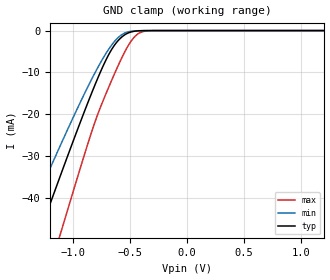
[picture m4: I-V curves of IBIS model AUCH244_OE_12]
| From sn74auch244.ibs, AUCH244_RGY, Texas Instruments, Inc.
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[Model]   AUCH244_OE_12
Model_type  Input
Vinl=0.385
Vinh=0.845
| variable   typ   min   max
C_comp   2.58pF   2.16pF   2.97pF
[Temperature Range]   40   100   -40
| Ambient temperature   25   85   -40
[Voltage range]   1.2   1.1   1.3
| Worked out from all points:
|   GND clamp passes 1 mA (typ) near -0.55 V on its own axis
[GND Clamp]
| AUCH244_OE_12
|   Voltage   I(typ)   I(min)   I(max)
-3.6V     -226.6mA   -190.3mA   -271.8mA
-1.47V    -61.86mA   -49.74mA   -81.22mA
-1.425V   -58.42mA   -46.89mA   -77.15mA
-1.295V   -48.52mA   -38.74mA   -65.35mA
-1.13V    -36.11mA   -28.6mA    -50.37mA
-1.09V    -33.13mA   -26.19mA   -46.74mA
-835mV    -14.83mA   -11.55mA   -24.08mA
-690mV    -5.892mA   -4.567mA   -13.74mA
-570mV    -1.488mA   -943.5uA   -6.381mA
-435mV    -83.64uA   -40.42uA   -873uA
-295mV    -1.276uA   -867.5nA   -9.761uA
1.2V      133.3pA    224.2pA    123.7pA
